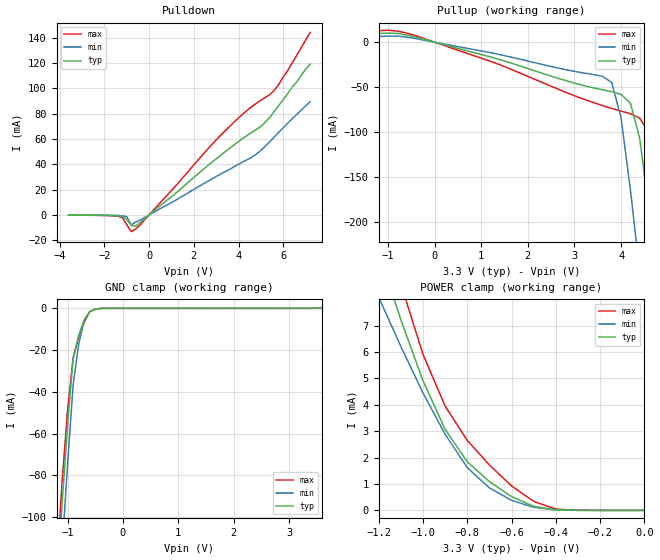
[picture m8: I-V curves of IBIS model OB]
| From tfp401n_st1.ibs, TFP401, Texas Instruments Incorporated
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|   OUTPUT  MODEL
[Model]   OB
Model_type   3-state
| Signals   QE, QO, HSYNC, VSYNC, DE
| variable   typ   min   max
C_comp   2pF   NA   NA
|   typ   min   max
[Temperature Range] 25.0   70.0   0.0
[Voltage range]   3.3V   3.0V   3.6V
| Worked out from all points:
|   slope of the pulldown table from 0 to 0.495 V, typ, clamps not added: 68.3 ohm
|   slope of the pullup table from 0 to 0.495 V, typ, clamps not added: 72.4 ohm
|   GND clamp passes 1 mA (typ) near -0.56 V on its own axis
|   POWER clamp passes 1 mA (typ) near -0.68 V on its own axis
[GND_clamp]
|Voltage   I(typ)   I(min)   I(max)
-3.6V     -1.31A     -1.33A     -1.29A
-1.2V     -137mA     -160mA     -125mA
-1.1V     -93.7mA    -116mA     -83.3mA
-1V       -55.7mA    -74.4mA    -48.7mA
-900mV    -24.2mA    -36.7mA    -23.6mA
-800mV    -12.9mA    -17.2mA    -13.8mA
-700mV    -5.55mA    -5.81mA    -6.57mA
-600mV    -1.42mA    -1.58mA    -1.64mA
-500mV    -415uA     -488uA     -470uA
-400mV    -33.7uA    -58.2uA    -32.4uA
3.3V      248pA      1.48uA     197pA
3.6V      729nA      378uA      240pA
[Power_clamp]
|Note that the [Power_clamp] voltage table is referenced to Vcc
|and is calculated using Vtable=Vcc-Vmeasured.
|Voltage   I(typ)   I(min)   I(max)
-3.3V     71.1mA     50.7mA     91.2mA
-1.2V     9.79mA     8.07mA     11.7mA
-1.1V     7.22mA     6.21mA     8.58mA
-1V       4.91mA     4.45mA     5.91mA
-900mV    3.07mA     2.88mA     3.95mA
-800mV    1.84mA     1.62mA     2.65mA
-700mV    1.09mA     850uA      1.72mA
-600mV    524uA      380uA      926uA
-500mV    152uA      117uA      341uA
-400mV    18uA       14.5uA     47.1uA
-300mV    1.13uA     1.43uA     3.52uA
0V        124pA      197pA      131pA
[Pulldown]
|Voltage   I(typ)   I(min)   I(max)
-3.6V     -122uA     -84.2uA    -158uA
-1.4V     -589uA     -316uA     -898uA
-1.2V     -1.39mA    -774uA     -2.18mA
-1V       -3.46mA    -1.38mA    -7.72mA
-800mV    -8.21mA    -7.72mA    -13.2mA
-600mV    -8.98mA    -5.74mA    -11.2mA
3.4V      49.9mA     34.2mA     66.4mA
4.8V      67.5mA     48mA       88.2mA
5.2V      73.2mA     54.3mA     92.8mA
5.6V      81.7mA     61.6mA     98.5mA
6.2V      95.9mA     72.5mA     114mA
7.2V      119mA      89.3mA     144mA
[Pullup]
|Note that the [Pullup] voltage table is referenced to Vcc
|and is calculated using Vtable=Vcc-Vmeasured.
|Voltage   I(typ)   I(min)   I(max)
-3.2V     2.58mA     2.04mA     3.19mA
-800mV    9.74mA     6.71mA     12.4mA
1.2V      -16.4mA    -11.6mA    -21.3mA
3.6V      -52.9mA    -37.9mA    -70.5mA
3.8V      -55mA      -44.8mA    -73.6mA
4V        -58.1mA    -84.2mA    -76.6mA
4.2V      -67.8mA    -164mA     -79.4mA
4.4V      -107mA     -255mA     -84.5mA
4.6V      -188mA     -349mA     -101mA
4.8V      -279mA     -445mA     -142mA
5V        -374mA     -542mA     -223mA
6.6V      -1.16A     -1.33A     -998mA
[Ramp]
|   typ   min   max
dV/dt_r   1.95v/0.84ns   1.76v/1.29ns   2.14v/0.57ns
dV/dt_f   1.95v/0.64ns   1.77v/1.02ns   2.14v/0.41ns
R_load = 5K
